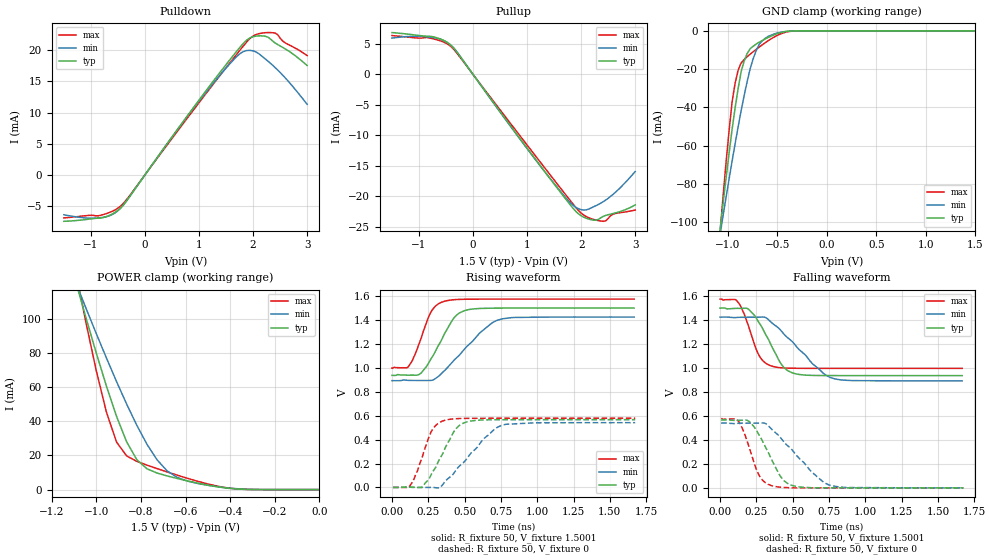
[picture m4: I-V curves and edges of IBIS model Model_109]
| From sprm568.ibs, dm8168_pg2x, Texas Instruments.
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| Model based on original model for BSHTLTCSCDVGPBFZ
|   Sub model SLOWEST_5MA_5PER_1P5
[model]   Model_109
|[Description]  [1.5V-3-STATE-X-SLOWEST:5MA, IND, 5%]
|   Slowest slew rate (SR[1:0] = "11"), 1.60 * RExt = 0.625 * Iout
|   (I[2:0] = "000"), 5mA nominal with Rext = 50R, ,Industrial
|   temperature range (-40C to 125C, 25C nominal),5% power supply
|   tolerance
|[Input Load]
|[Output Drive] SLOWEST:5MA
|Voltage   1.5V
|Mode   3-STATE
Model_type   3-state
Polarity   Non-Inverting
Enable   Active-Low
Cref =  15.0000pF
Rref =  100.0000M
Vref =  0V
Vmeas =  0.75005
C_comp   1.5249p   1.4275p   1.6205p
[Model Spec]
[Temperature Range]   25   125   -40
[Voltage Range]   1.5   1.425   1.575
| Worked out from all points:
|   slope of the pulldown table from 0 to 0.225 V, typ, clamps not added: 81.7 ohm
|   slope of the pullup table from 0 to 0.225 V, typ, clamps not added: 81.7 ohm
|   GND clamp passes 1 mA (typ) near -0.47 V on its own axis
|   POWER clamp passes 1 mA (typ) near -0.42 V on its own axis
|   rising waveform, R_fixture 50, V_fixture 1.5001: 20-80 % time 153ps typ, 251ps min, 106ps max; typ from 0.937 V to 1.5 V
|   rising waveform, R_fixture 50, V_fixture 0: 20-80 % time 147ps typ, 239ps min, 102ps max; typ from 0 V to 0.566 V
|   falling waveform, R_fixture 50, V_fixture 1.5001: 20-80 % time 149ps typ, 258ps min, 102ps max; typ from 1.5 V to 0.937 V
|   falling waveform, R_fixture 50, V_fixture 0: 20-80 % time 144ps typ, 247ps min, 99.4ps max; typ from 0.566 V to 0 V
[POWER_clamp]
-1.5V     321.7mA    260.6mA    415.9mA
-1.076V   114.2mA    115.8mA    116.9mA
-1.061V   107.2mA    110.9mA    107.1mA
-954.6mV  60.59mA    77.06mA    45.35mA
-909.2mV  42.85mA    63.21mA    27.81mA
-863.7mV  27.9mA     49.99mA    19.69mA
-818.2mV  17.49mA    37.63mA    16.52mA
-772.8mV  12.19mA    26.53mA    14.33mA
-681.9mV  7.985mA    10.89mA    10.33mA
-590.9mV  5.094mA    4.955mA    6.6mA
-363.7mV  298.5uA    465.2uA    297.6uA
0V        1.518nA    24.08nA    367.8pA
[Pulldown]
-1.5V     -7.45mA    -6.4mA     -6.9mA
-863.7mV  -6.95mA    -6.903mA   -6.565mA
-500mV    -5.682mA   -5.758mA   -5.339mA
-318.2mV  -3.897mA   -3.924mA   -3.728mA
1.046V    12.53mA    12.35mA    12.1mA
1.591V    18.69mA    18.02mA    18.2mA
1.818V    21.09mA    19.78mA    20.66mA
1.955V    22.02mA    19.97mA    21.99mA
2.091V    22.3mA     19.54mA    22.62mA
2.273V    22.11mA    18.26mA    22.84mA
2.364V    21.46mA    17.58mA    22.81mA
3V        17.55mA    11.32mA    19.14mA
[Pullup]
-1.5V     6.87mA     5.96mA     6.38mA
-818.2mV  6.271mA    6.141mA    6.005mA
-590.9mV  5.763mA    5.741mA    5.469mA
-409.1mV  4.8mA      4.791mA    4.587mA
1.227V    -14.81mA   -14.84mA   -14.21mA
1.727V    -20.63mA   -20.37mA   -19.92mA
1.909V    -22.57mA   -21.88mA   -21.95mA
2.046V    -23.45mA   -22.28mA   -23.09mA
2.227V    -23.93mA   -21.76mA   -23.82mA
2.409V    -23.32mA   -20.9mA    -24.13mA
2.591V    -22.85mA   -19.7mA    -22.97mA
3V        -21.43mA   -15.95mA   -22.28mA
[GND_clamp]
-1.5V     -310.1mA   -250.5mA   -402.5mA
-1.076V   -103.6mA   -106.2mA   -105.2mA
-1.046V   -89.81mA   -96.36mA   -86.02mA
-954.6mV  -51.22mA   -67.87mA   -36.88mA
-924.3mV  -40.08mA   -58.86mA   -27.29mA
-863.7mV  -21.24mA   -41.56mA   -16.73mA
-833.4mV  -15.8mA    -33.75mA   -15.03mA
-772.8mV  -9.345mA   -19.75mA   -12.19mA
-712.2mV  -6.928mA   -10.35mA   -9.704mA
-621.3mV  -4.261mA   -3.896mA   -6.225mA
-409.1mV  -337.1uA   -289.1uA   -618.9uA
1.5V      1.518nA    257.2nA    299pA
[Ramp]
dV/dt_f   0.450848/0.21618379n   0.426056/0.36102103n   0.462408/0.15905928n
dV/dt_r 0.45461936/0.21202598n 0.43623312/0.33979347n 0.46290425/0.15633101n
R_load = 50
[Rising Waveform]
R_fixture = 50
V_fixture = 1.5001
V_fixture_min = 1.425
V_fixture_max = 1.575
0s        937.3mV    893.3mV    997.8mV
109.4ps   938.9mV    895.7mV    1.006V
143.6ps   939.3mV    894.8mV    1.07V
196.9ps   953.3mV    894.1mV    1.234V
273.6ps   1.084V     895.9mV    1.477V
360.1ps   1.281V     975.1mV    1.557V
467.8ps   1.462V     1.112V     1.573V
604ps     1.497V     1.292V     1.575V
758.3ps   1.5V       1.41V      1.575V
1.667ns   1.5V       1.425V     1.575V
[Rising Waveform]
R_fixture = 50
V_fixture = 0
V_fixture_min = 0
V_fixture_max = 0
7.64ps    0V         0V         0V
118.7ps   2.057mV    2.409mV    5.352mV
206.1ps   0V         0V         244.2mV
279ps     127.2mV    0V         484mV
360.9ps   314mV      42.26mV    560.6mV
429.3ps   471.9mV    124mV      573.8mV
478.3ps   529.6mV    193.5mV    576.7mV
638.1ps   564.6mV    413.7mV    578.4mV
751.7ps   566.2mV    517.3mV    578.5mV
1.674ns   566.5mV    541.4mV    578.6mV
[Falling Waveform]
R_fixture = 50
V_fixture = 1.5001
V_fixture_min = 1.425
V_fixture_max = 1.575
0s        1.5V       1.424V     1.575V
112.1ps   1.498V     1.421V     1.565V
195.7ps   1.491V     1.423V     1.352V
271.9ps   1.372V     1.424V     1.099V
364.3ps   1.16V      1.369V     1.013V
431.7ps   1.016V     1.295V     1.001V
496.4ps   959.8mV    1.222V     998.1mV
642.2ps   938mV      1.029V     997.1mV
788.6ps   936.7mV    909.5mV    997mV
1.667ns   936.6mV    892.7mV    997mV
[Falling Waveform]
R_fixture = 50
V_fixture = 0
V_fixture_min = 0
V_fixture_max = 0
7.64ps    565.5mV    540.5mV    577.7mV
130.4ps   563.8mV    539mV      549.8mV
198.8ps   555.2mV    540mV      345.9mV
264.4ps   450.4mV    540.2mV    115.8mV
352.4ps   243.3mV    493.3mV    18.94mV
420ps     89.31mV    413.7mV    4.909mV
479.8ps   27.92mV    337mV      0V
633.8ps   0V         129.7mV    0V
763ps     0V         19.34mV    0V
1.674ns   0V         0V         0V
